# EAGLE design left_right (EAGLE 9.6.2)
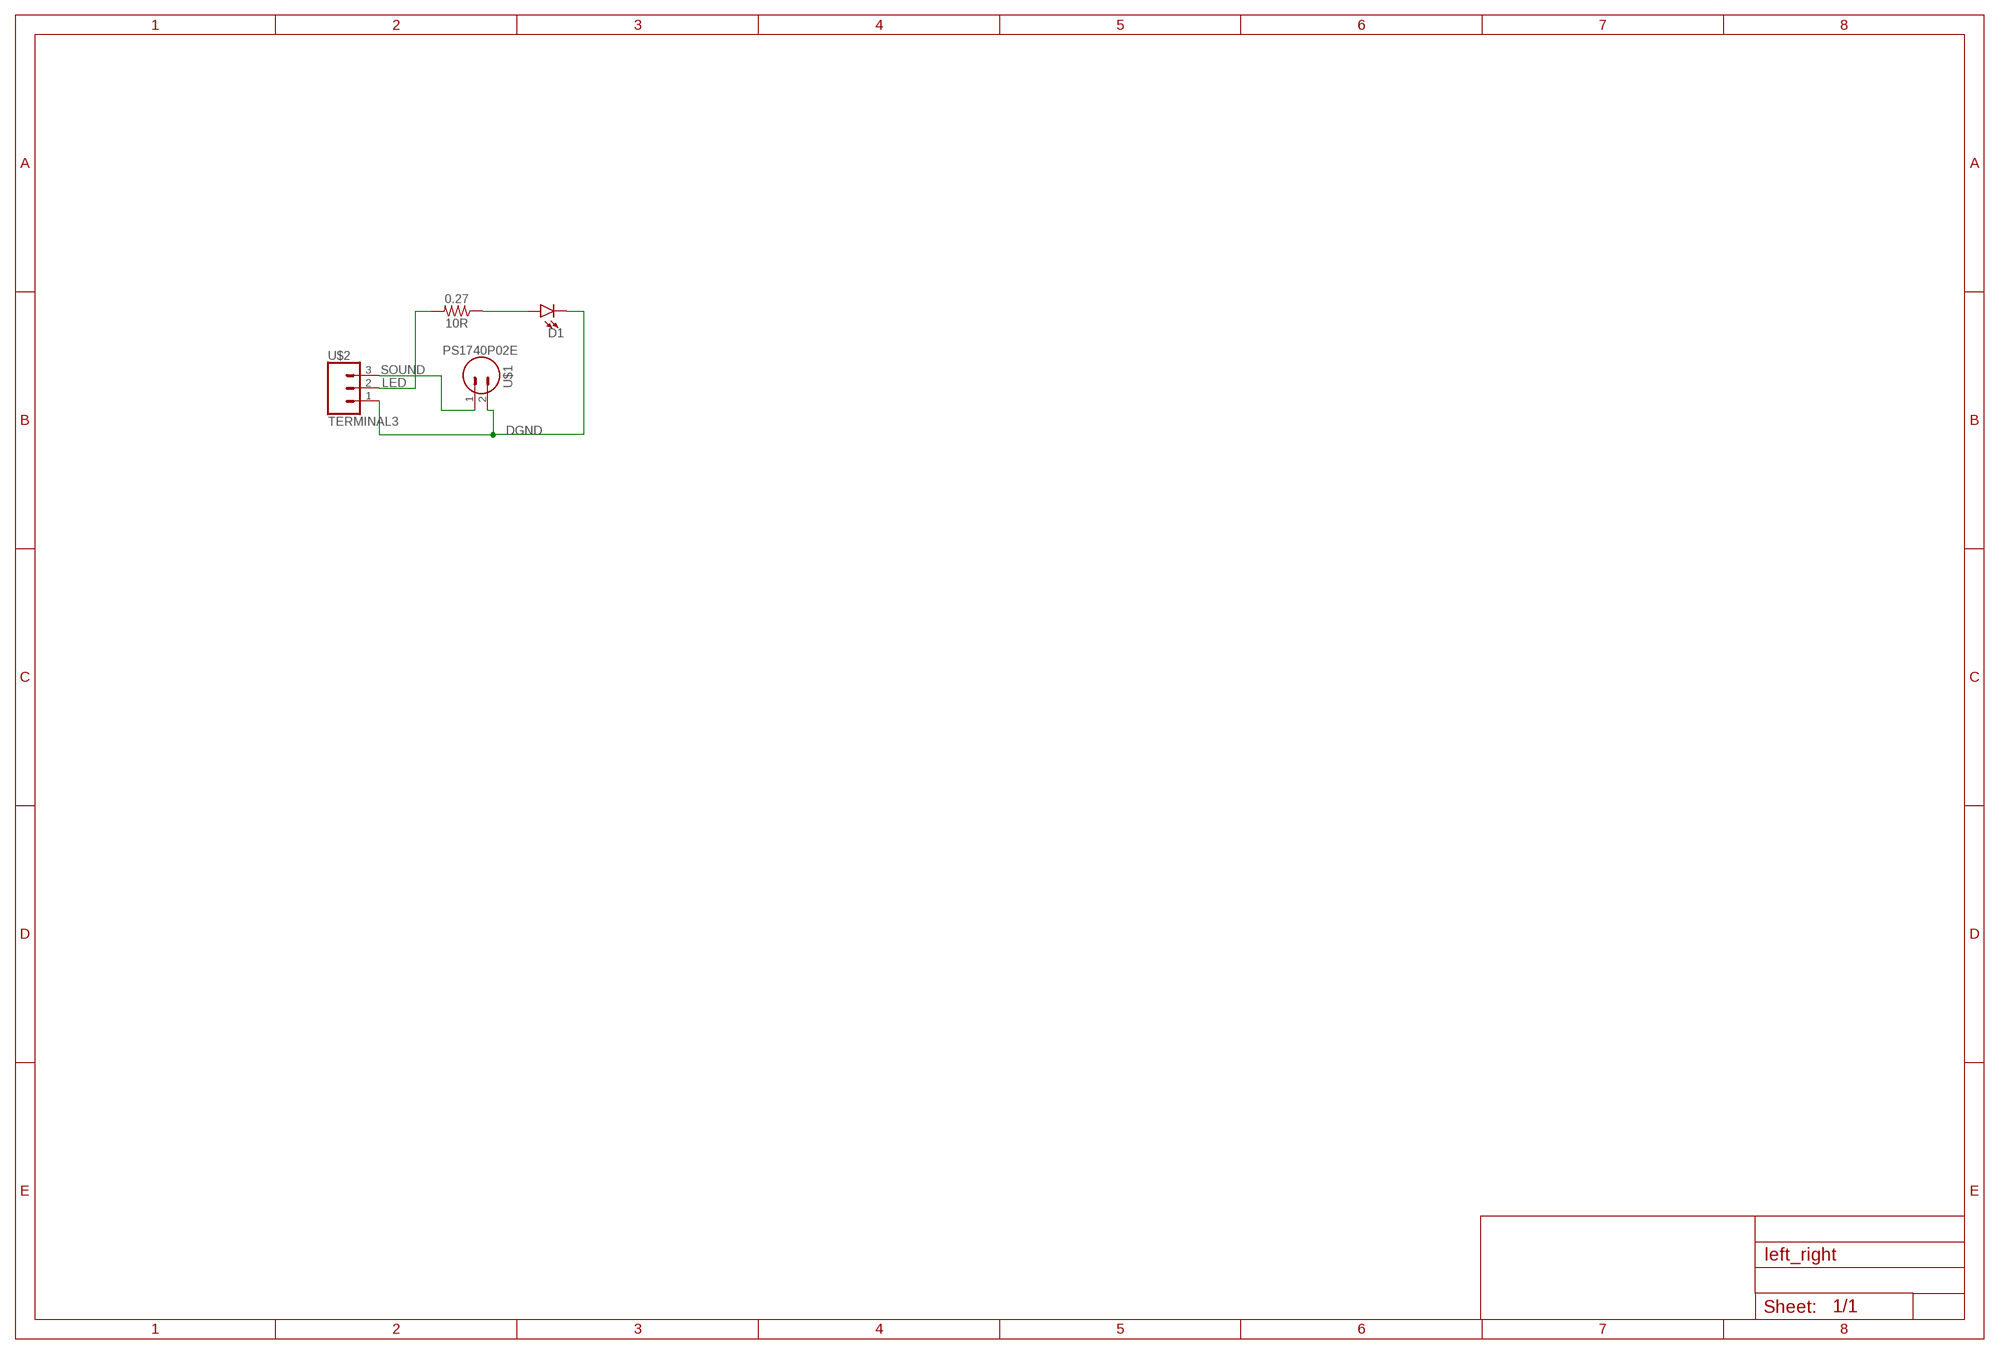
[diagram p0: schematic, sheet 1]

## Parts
10R  0.27  0.27OHM-0603-1/10W-1%  [0603]
D1  LED-35281206  [3528]
U$1  PS1740P02E  [PS1740]
U$2  TERMINAL3  [1X3]

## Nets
DGND: D1.C U$1.2 U$2.1
LED: 10R.2 U$2.2
N$2: 10R.1 D1.A
SOUND: U$1.1 U$2.3

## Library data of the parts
10R = SparkFun-Resistors:0.27OHM: 0.27Ω resistor; PROD_ID: RES-08787
D1 = habits:LED-3528: LED (Generic)
U$1 = habits:PS1740P02E
U$2 = habits:TERMINAL3

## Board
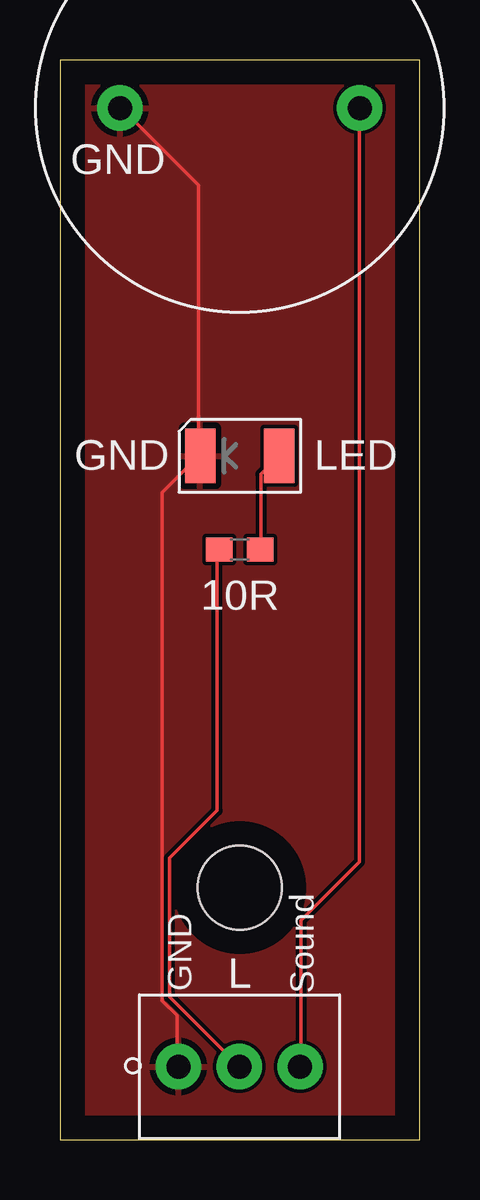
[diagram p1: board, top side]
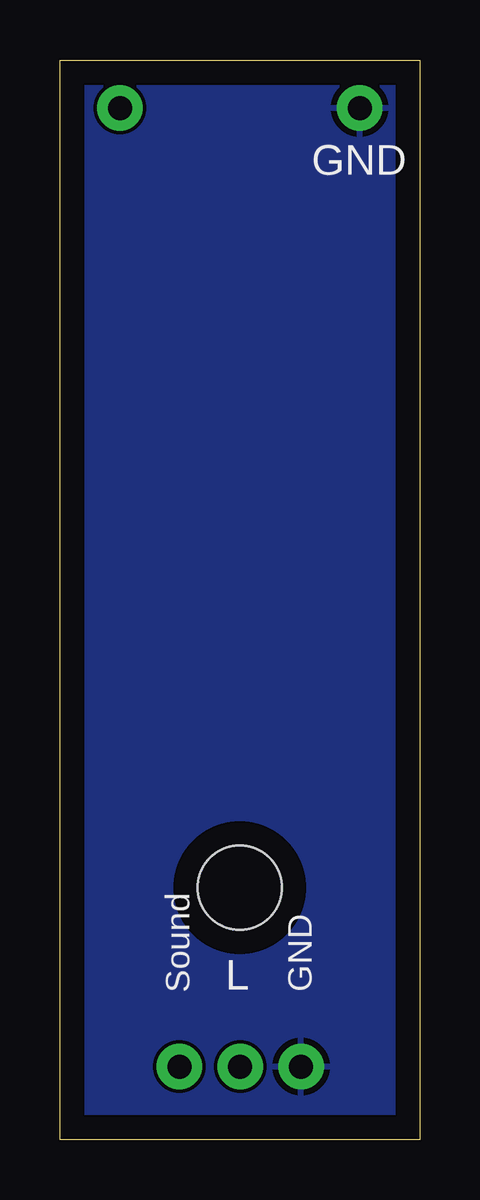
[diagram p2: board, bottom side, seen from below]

Size 15 x 45 mm. Coordinates in mm from the lower left corner, seen from the top.
Outline: 0,0 15,0 15,45 0,45 0,0
Copper layers (1*16): Top 0.035mm / dielectric 1.5mm / Bottom 0.035mm
Design rules "default": minimum track width 6mil, minimum drill 0.35mm, track to track 6mil, track to pad 6mil, pad to pad 6mil, via to via 6mil, smd to smd 6mil, copper to edge 40mil, drill to drill 6mil, minimum pad ring 10mil, minimum via ring 8mil, stop-mask expansion 4mil, vias tented up to drill 0mil, thermal gap 10mil
Holes 3.5 mm at 7.5,10.5

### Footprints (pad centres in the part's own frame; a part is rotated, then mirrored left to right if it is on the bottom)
0603 = smd 1.1 x 1: 1 -0.85,0; 2 0.85,0
3528 = smd 1.27 x 2.286: A -1.651,0; C 1.651,0
PS1740 = drill 1 pad 1.9: 1 0,0; 2 10,0
1X3 = drill 1 pad 1.9: 1 0,0; 2 2.54,0; 3 5.08,0

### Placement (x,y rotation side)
10R  7.5,24.6 180 top
D1  7.5,28.5 180 top
U$1  12.5,43 180 top
U$2  4.94,3.04 0 top

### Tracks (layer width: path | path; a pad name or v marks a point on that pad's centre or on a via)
DGND
  Top 0.152: U$1.2 2.59,42.98 5.79,39.78 5.79,28.65 D1.C 5.79,28.5 4.27,26.98 4.27,5.79 4.88,5.18 4.88,3.05 U$2.1
  pour Top: 0,0 15,0 15,45 0,45
  pour Bottom: 0,0 15,0 15,45 0,45
LED
  Top 0.152: 10R.2 6.55,24.54 6.55,13.72 4.57,11.73 4.57,5.94 7.47,3.05 U$2.2
N$2
  Top 0.152: 10R.1 8.38,24.69 8.38,27.74 D1.A
SOUND
  Top 0.152: U$2.3 10.06,3.05 10.06,9.14 12.5,11.58 12.5,42.98 U$1.1

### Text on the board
tPlace: GND | GND | LED | GND | L | Sound
bPlace: GND | Sound | GND | L

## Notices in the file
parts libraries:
SparkFun-Resistors: Licensing: Creative Commons ShareAlike 4.0 International - https://creativecommons.org/licenses/by-sa/4.0
